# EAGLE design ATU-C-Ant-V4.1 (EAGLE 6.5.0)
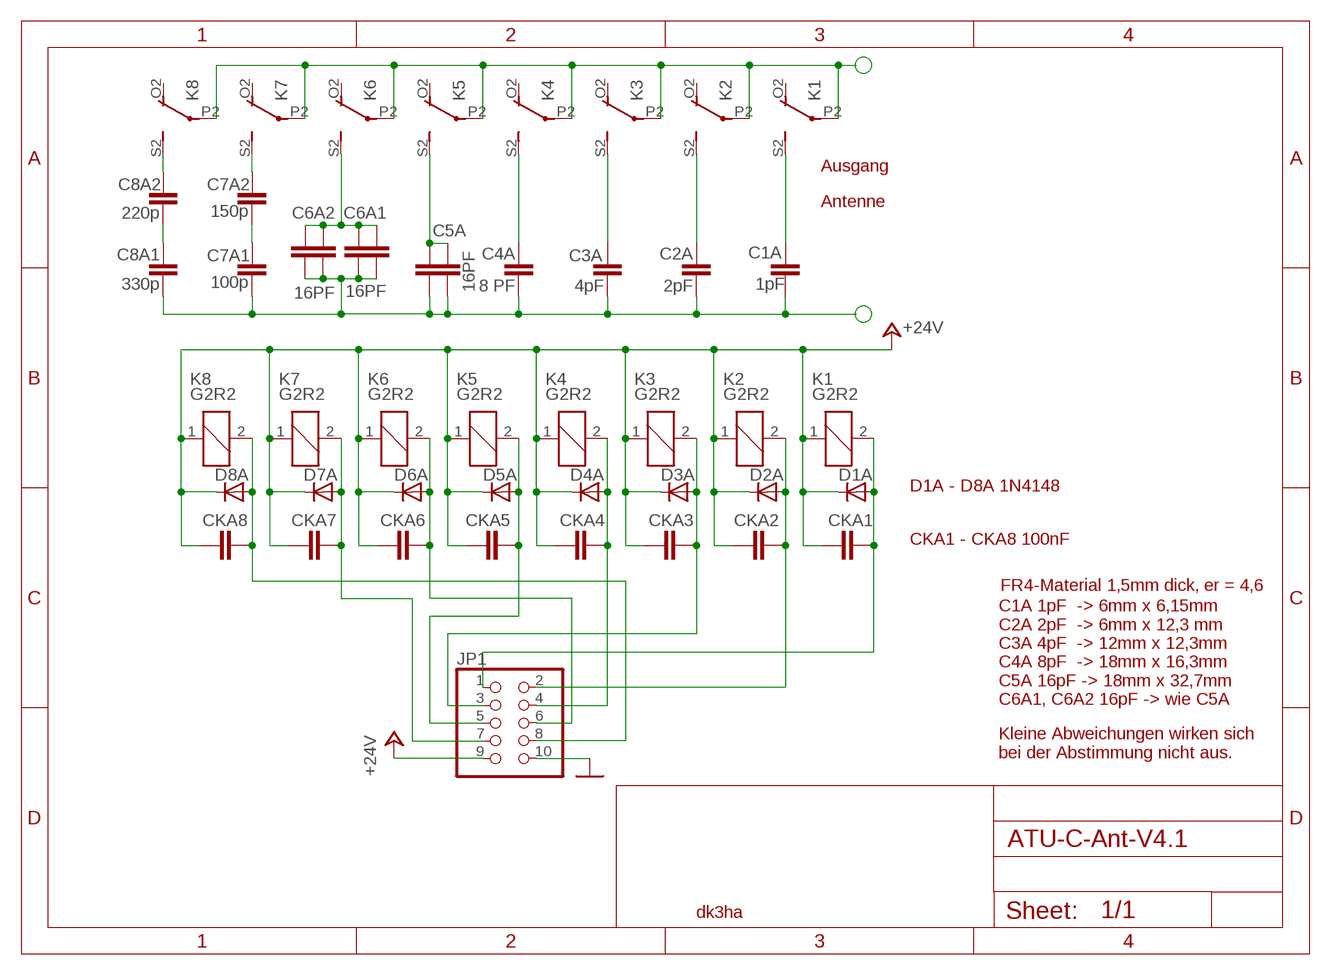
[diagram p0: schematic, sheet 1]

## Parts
C1A  1pF  1PF-CU-DS-ER4,6-D1,5  [1PF-ER4.6-DS-1,5]
C2A  2pF  2PF-CU-DS-ER4,6-D1,5  [2PF-ER4.6-DS-1,5]
C3A  4pF  4PF-CU-DS-ER4,6-D1,5  [4PF-ER4.6-DS-1,5]
C4A  8 PF  8PF-CU-DS-ER4,6-D1,5  [8PF-ER4.6-DS-1,5]
C5A  16PF  16PF-CU-DS-ER4,6-D1,5  [16PF-ER4.6-DS-1,5]
C6A1  16PF  16PF-CU-DS-ER4,6-D1,5  [16PF-ER4.6-DS-1,5]
C6A2  16PF  16PF-CU-DS-ER4,6-D1,5  [16PF-ER4.6-DS-1,5]
C7A1  100p  C15/5  [C15B5]
C7A2  150p  C15/5  [C15B5]
C8A1  330p  C15/5  [C15B5]
C8A2  220p  C15/5  [C15B5]
CKA1  C-EUC1206  [C1206]
CKA2  C-EUC1206  [C1206]
CKA3  C-EUC1206  [C1206]
CKA4  C-EUC1206  [C1206]
CKA5  C-EUC1206  [C1206]
CKA6  C-EUC1206  [C1206]
CKA7  C-EUC1206  [C1206]
CKA8  C-EUC1206  [C1206]
D1A  DIODE-MINIMELF  [MINIMELF]
D2A  DIODE-MINIMELF  [MINIMELF]
D3A  DIODE-MINIMELF  [MINIMELF]
D4A  DIODE-MINIMELF  [MINIMELF]
D5A  DIODE-MINIMELF  [MINIMELF]
D6A  DIODE-MINIMELF  [MINIMELF]
D7A  DIODE-MINIMELF  [MINIMELF]
D8A  DIODE-MINIMELF  [MINIMELF]
JP1  PINHD-2X5  [2X05]
K1  G2R2  [G2R2]
K2  G2R2  [G2R2]
K3  G2R2  [G2R2]
K4  G2R2  [G2R2]
K5  G2R2  [G2R2]
K6  G2R2  [G2R2]
K7  G2R2  [G2R2]
K8  G2R2  [G2R2]

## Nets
+24V: CKA1.1 CKA2.1 CKA3.1 CKA4.1 CKA5.1 CKA6.1 CKA7.1 CKA8.1 D1A.C D2A.C D3A.C D4A.C D5A.C D6A.C D7A.C D8A.C JP1.9 K1.1 K2.1 K3.1 K4.1 K5.1 K6.1 K7.1 K8.1
GND: JP1.10
LSP2: C1A.P$1 C2A.P$1 C3A.P$1 C4A.P$1 C5A.P$2 C5A.P$4 C6A1.P$2 C6A1.P$4 C6A2.P$2 C6A2.P$4 C7A1.2 C8A1.2
N$1: C6A1.P$1 C6A1.P$3 C6A2.P$1 C6A2.P$3 K6.S2(3:S)
N$3: C7A1.1 C7A2.1
N$4: C8A2.1 K8.S2(3:S)
N$5: C8A1.1 C8A2.2
N$6: C7A2.2 K7.S2(3:S)
N$7: C4A.P$2 K4.S2(3:S)
N$8: CKA1.2 D1A.A JP1.1 K1.2
N$9: K1.P2(3:P) K2.P2(3:P) K3.P2(3:P) K4.P2(3:P) K5.P2(3:P) K6.P2(3:P) K7.P2(3:P) K8.P2(3:P)
N$10: C3A.P$2 K3.S2(3:S)
N$11: CKA2.2 D2A.A JP1.2 K2.2
N$12: C2A.P$2 K2.S2(3:S)
N$13: CKA3.2 D3A.A JP1.3 K3.2
N$14: C1A.P$2 K1.S2(3:S)
N$15: CKA4.2 D4A.A JP1.4 K4.2
N$20: CKA6.2 D6A.A JP1.6 K6.2
N$22: C5A.P$1 C5A.P$3 K5.S2(3:S)
N$26: CKA7.2 D7A.A JP1.7 K7.2
N$28: CKA8.2 D8A.A JP1.8 K8.2
N$A5: CKA5.2 D5A.A JP1.5 K5.2
Unconnected: K1.O1(2:O) K1.O2(3:O) K1.P1(2:P) K1.S1(2:S) K2.O1(2:O) K2.O2(3:O) K2.P1(2:P) K2.S1(2:S) K3.O1(2:O) K3.O2(3:O) K3.P1(2:P) K3.S1(2:S) K4.O1(2:O) K4.O2(3:O) K4.P1(2:P) K4.S1(2:S) K5.O1(2:O) K5.O2(3:O) K5.P1(2:P) K5.S1(2:S) K6.O1(2:O) K6.O2(3:O) K6.P1(2:P) K6.S1(2:S) K7.O1(2:O) K7.O2(3:O) K7.P1(2:P) K7.S1(2:S) K8.O1(2:O) K8.O2(3:O) K8.P1(2:P) K8.S1(2:S)

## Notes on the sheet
- Ausgang
- Antenne
- D1A - D8A 1N4148
- CKA1 - CKA8 100nF
- FR4-Material 1,5mm dick, er = 4,6
- C1A 1pF  -> 6mm x 6,15mm
  C2A 2pF  -> 6mm x 12,3 mm
  C3A 4pF  -> 12mm x 12,3mm
  C4A 8pF  -> 18mm x 16,3mm
  C5A 16pF -> 18mm x 32,7mm
  C6A1, C6A2 16pF -> wie C5A
- Kleine Abweichungen wirken sich
  bei der Abstimmung nicht aus.
- dk3ha

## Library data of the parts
C1A = dk3ha-2020:1PF-CU-DS-ER4,6-D1,5: C doppelseitig Cu, d=1,5mm, Epoxy er=4,6 (Bungard), 1 pF, Maße 6,2mm x 6mm
C2A = dk3ha-2020:2PF-CU-DS-ER4,6-D1,5: C doppelseitig Cu, d=1,5mm, Epoxy er=4,6 (Bungard), 2 pF, Maße 12,3mm x 6mm
C3A = dk3ha-2020:4PF-CU-DS-ER4,6-D1,5: C doppelseitig Cu, d=1,5mm, Epoxy er=4,6 (Bungard), 4 pF, Maße 12,3mm x 12mm
C4A = dk3ha-2020:8PF-CU-DS-ER4,6-D1,5: C doppelseitig Cu, d=1,5mm, Epoxy er=4,6 (Bungard), 8 pF, Maße 16,4mm x 18mm
C5A C6A1 C6A2 = dk3ha-2020:16PF-CU-DS-ER4,6-D1,5: C doppelseitig Cu, d=1,5mm, Epoxy er=4,6 (Bungard), 16 pF, Maße 32,8mm x 18mm
C7A1 C7A2 C8A1 C8A2 = capacitor-wima:C: CAPACITOR
CKA1-CKA8 = rcl:C-EU: CAPACITOR, European symbol
D1A D2A D3A D4A D5A D6A D7A D8A = diode:DIODE-: DIODE
JP1 = pinhead+:PINHD-2X5: PIN HEADER
K1-K8 = relay:G2R2: RELAY 2 x switch, Omron; MF: OMRON COMPONENTS USA; MPN: G2R-2-DC6; OC_FARNELL: unknown; OC_NEWARK: 89C5317

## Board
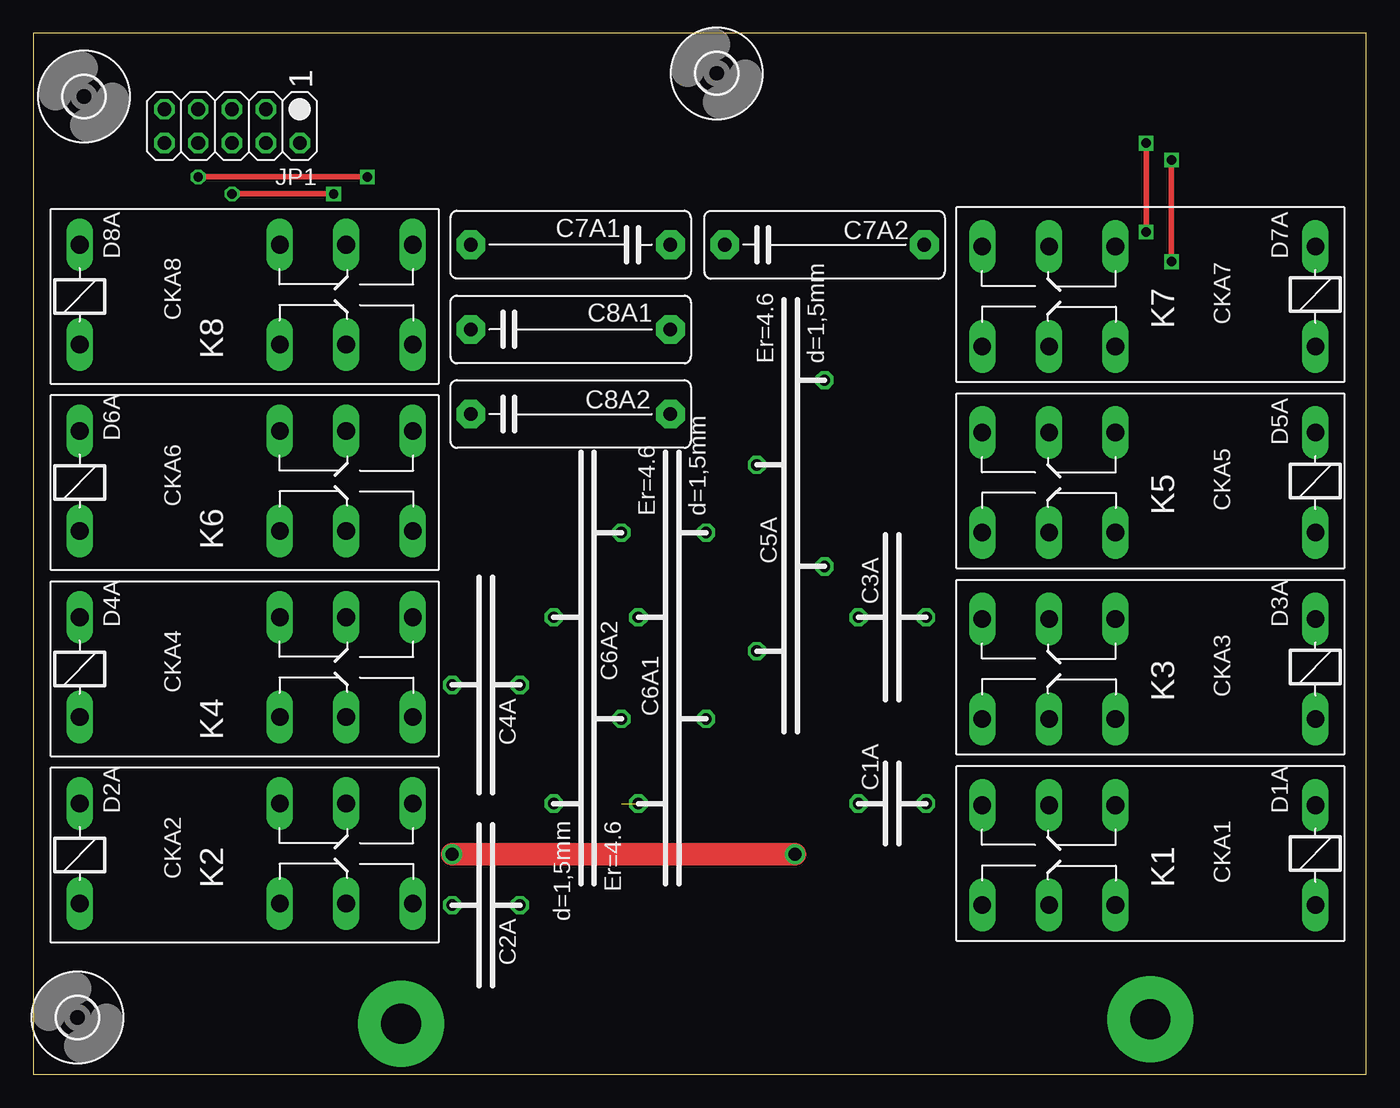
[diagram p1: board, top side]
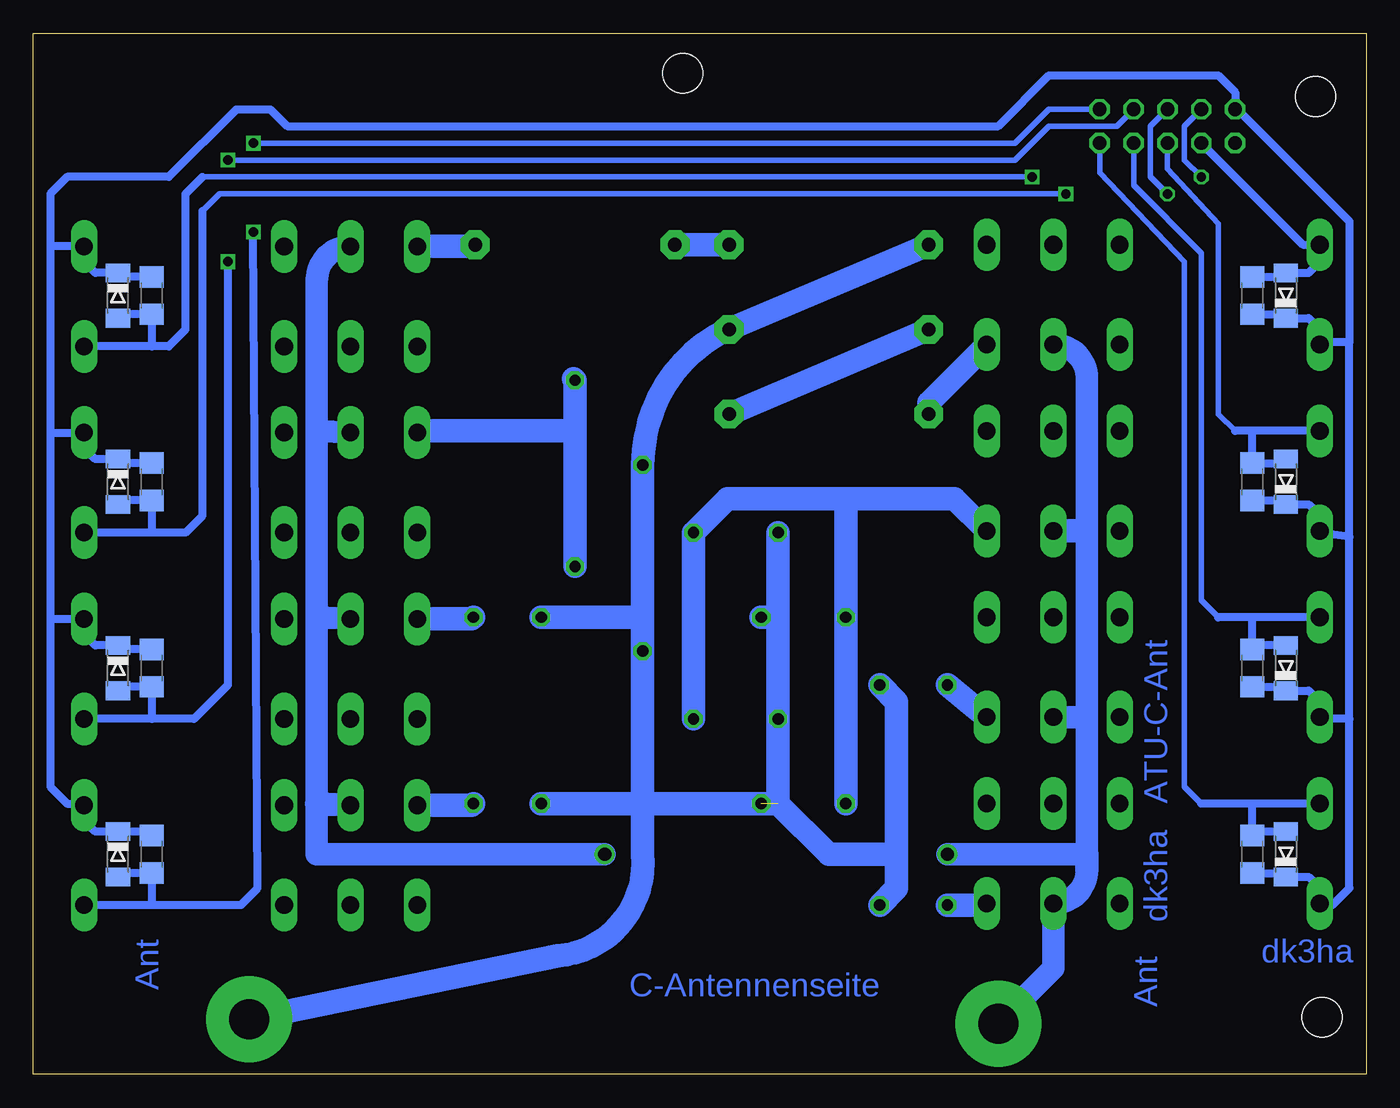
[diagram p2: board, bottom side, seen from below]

Size 100 x 78.08 mm. Coordinates in mm from the lower left corner, seen from the top.
Outline: 100,0 100,78.08 0,78.08 0,0 100,0
Copper layers (1*16): Top 0.035mm / dielectric 1.5mm / Bottom 0.035mm
Design rules "default": minimum track width 10mil, minimum drill 24mil, track to track 8mil, track to pad 8mil, pad to pad 8mil, via to via 8mil, smd to smd 8mil, copper to edge 40mil, drill to drill 8mil, minimum pad ring 10mil, minimum via ring 8mil, stop-mask expansion 4mil, vias tented up to drill 0mil, thermal gap 10mil

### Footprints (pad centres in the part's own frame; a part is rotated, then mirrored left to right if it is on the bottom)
1PF-ER4.6-DS-1,5 = drill 0.85 octagon: P$1 -2.54,0; P$2 2.54,0
2PF-ER4.6-DS-1,5 = drill 0.85 octagon: P$1 -2.54,0; P$2 2.54,0
4PF-ER4.6-DS-1,5 = drill 0.85 octagon: P$1 -2.54,0; P$2 2.54,0
8PF-ER4.6-DS-1,5 = drill 0.85 octagon: P$1 -2.54,0; P$2 2.54,0
16PF-ER4.6-DS-1,5 = drill 0.85 octagon: P$1 2.54,10.16; P$2 -2.54,3.81; P$3 2.54,-3.81; P$4 -2.54,-10.16
C15B5 = drill 1.016 pad 2.159 octagon: 1 -7.493,0; 2 7.493,0
C1206 = smd 1.6 x 1.8: 1 -1.4,0; 2 1.4,0
MINIMELF = smd 1.4 x 1.8: A 1.7,0; C -1.7,0
2X05 = drill 1.016 octagon: 1 -5.08,-1.27; 2 -5.08,1.27; 3 -2.54,-1.27; 4 -2.54,1.27; 5 0,-1.27; 6 0,1.27; 7 2.54,-1.27; 8 2.54,1.27; 9 5.08,-1.27; 10 5.08,1.27
G2R2 = drill 1.321 long: 1 -2.54,-3.683; 2 -2.54,3.81; O1 12.471,3.81; O2 12.471,-3.683; P1 17.45,3.81; P2 17.45,-3.683; S1 22.454,3.81; S2 22.454,-3.683
3,0 = hole 3: 0,0

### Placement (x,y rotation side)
C1A  64.44,20.32 0 top
C2A  33.96,12.7 180 top
C3A  64.44,34.29 0 top
C4A  33.96,29.21 180 top
C5A  56.82,41.91 0 top
C6A1  47.93,30.48 0 top
C6A2  41.58,30.48 180 top
C7A1  40.31,62.23 180 top
C7A2  59.36,62.23 0 top
C8A1  40.31,55.88 0 top
C8A2  40.31,49.53 0 top
CKA1  91.11,16.51 270 bottom
CKA2  8.56,16.51 90 bottom
CKA3  91.11,30.48 270 bottom
CKA4  8.56,30.48 90 bottom
CKA5  91.11,44.45 270 bottom
CKA6  8.56,44.45 90 bottom
CKA7  91.11,58.42 270 bottom
CKA8  8.56,58.42 90 bottom
D1A  93.65,16.51 270 bottom
D2A  6.02,16.51 90 bottom
D3A  93.65,30.48 270 bottom
D4A  6.02,30.48 90 bottom
D5A  93.65,44.45 270 bottom
D6A  6.02,44.45 90 bottom
D7A  93.65,58.42 270 bottom
D8A  6.02,58.42 90 bottom
JP1  14.91,71.12 180 top
K1  93.65,16.51 180 top
K2  6.02,16.51 0 top
K3  93.65,30.48 180 top
K4  6.02,30.48 0 top
K5  93.65,44.45 180 top
K6  6.02,44.45 0 top
K7  93.65,58.42 180 top
K8  6.02,58.42 0 top
U$1  [3,0]  3.8,73.34 90 top
U$2  [3,0]  3.32,4.29 90 top
U$3  [3,0]  51.26,75.09 90 top

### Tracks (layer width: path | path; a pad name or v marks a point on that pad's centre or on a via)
+24V
  Bottom 0.61: 98.73,34.16 K3.1 96.19,33.02 95.35,32.18 D3A.C 93.35,31.88 CKA3.1 | 98.73,48.13 K5.1 96.19,46.99 95.35,46.15 D5A.C 93.35,45.85 CKA5.1 | K2.1 3.48,12.7 | K4.1 3.48,26.67 | K6.1 3.48,40.64 | K8.1 3.48,54.61 | 1.26,26.67 1.26,13.97 2.53,12.7 3.61,12.7 K2.1 | 1.26,26.67 1.26,40.32 | 1.26,40.32 1.26,54.93 | 1.26,54.93 1.26,63.82 1.26,63.98 9.67,72.39 JP1.9 9.83,73.66 11.1,74.93 23.8,74.93 27.61,71.12 80.95,71.12 82.22,72.39 84.76,72.39 89.84,67.31 97.46,67.31 98.73,66.04 98.73,62.23 | 98.73,62.23 98.73,48.13 | 98.73,48.13 98.73,34.16 | 98.73,34.16 98.73,21.59 97.46,20.32 96.32,20.32 K1.1 96.19,19.05 95.35,18.21 D1A.C 91.11,18.21 CKA1.1 | 98.73,62.23 98.6,62.1 K7.1 96.19,60.96 95.35,60.12 D7A.C 93.35,59.82 CKA7.1 | 1.26,26.67 3.61,26.67 K4.1 | 1.26,40.32 3.61,40.64 K6.1 | 1.26,54.93 3.67,54.93 K8.1 | CKA2.1 6.32,15.11 D2A.C 4.32,14.81 3.48,13.97 K2.1 | CKA4.1 6.32,29.08 D4A.C 4.32,28.78 3.48,27.94 K4.1 | CKA6.1 6.32,43.05 D6A.C 4.32,42.75 3.48,41.91 K6.1 | CKA8.1 6.32,57.02 D8A.C 4.32,56.72 3.48,55.88 K8.1
LSP2  (via drill 3 pad 6.45)  (1 unrouted)
  Bottom 1.778: C1A.P$1 54.28,20.32 | C7A1.2 C8A1.2 47.93,55.88 arc-64 C5A.P$2 54.28,34.29 | 54.28,34.29 C5A.P$4 54.28,20.32 | C3A.P$1 54.28,34.29 | C4A.P$1 35.23,27.94 35.23,16.51 | 35.23,16.51 35.23,13.97 C2A.P$1 | C6A2.P$4 44.12,34.29 | 44.12,34.29 C6A2.P$2 44.12,20.32 | 44.12,20.32 40.31,16.51 35.23,16.51 | C6A1.P$2 44.12,34.29 | 54.28,20.32 44.12,20.32 | 54.28,20.32 54.28,16.51 arc90 60.63,8.89 v83.81,4.13
N$1
  Bottom 1.778: C6A1.P$3 C6A1.P$1 47.93,43.18 39.04,43.18 | 39.04,43.18 30.89,43.18 K6.S2 | 39.04,43.18 C6A2.P$3 C6A2.P$1
N$3
  Bottom 1.778: C7A1.1 C7A2.1
N$4
  Bottom 1.778: C8A2.1 32.82,50.39 K8.S2
N$5
  Bottom 1.778: C8A2.2 C8A1.1
N$6
  Bottom 1.778: K7.S2 67.11,62.1 66.98,62.23 C7A2.2
N$7
  Bottom 1.778: C4A.P$2 29.87,27.94 K4.S2
N$8  (via drill 0.7)
  Top 0.406: v83.49,63.18 v83.49,69.85
  Bottom 0.406: v83.49,69.85 26.34,69.85 23.8,72.39 JP1.1
  Bottom 0.61: v83.49,63.18 83.17,13.97 84.44,12.7 91.11,12.7 | 91.11,12.7 K1.2 | 91.11,12.7 CKA1.2 93.35,15.11 D1A.A
N$9  (via drill 1 pad 1.27, 3 pad 6.45)
  Top 1.676: v57.14,16.51 v31.42,16.51
  Bottom 1.524: 21.07,26.8 20.94,26.67 | 21.07,40.77 20.94,40.64 | K2.P2 23.67,12.83
  Bottom 1.676: K4.P2 21.07,26.8 | 78.73,48.26 78.73,59.58 arc90 K7.P2 | 78.73,48.26 78.73,34.29 | 78.73,34.29 78.73,20.32 78.73,16.51 v57.14,16.51 60.63,16.51 | v31.42,16.51 20.94,16.51 20.94,26.67 20.94,40.64 20.94,52.21 arc-90 K8.P2 | K3.P2 78.73,34.29 | K5.P2 78.73,48.26 | 20.94,15.35 arc90 K2.P2 23.47,7.95 v27.61,3.81
  Bottom 1.778: 20.94,16.51 20.94,15.35 | K6.P2 21.07,40.77 | K1.P2 78.73,20.32
N$10
  Bottom 1.778: K3.S2 67.11,34.16 C3A.P$2
N$11
  Bottom 0.406: JP1.2 19.99,67.63 13.64,60.96 13.64,21.59 12.37,20.32
  Bottom 0.61: K2.2 8.56,20.32 | 8.56,20.32 12.37,20.32 | 8.56,20.32 CKA2.2 8.26,18.21 D2A.A
N$12
  Bottom 1.778: C2A.P$2 28.6,12.7 K2.S2
N$13  (via drill 0.7)
  Top 0.406: v85.39,60.96 v85.39,68.58
  Bottom 0.406: v85.39,68.58 26.34,68.58 23.8,71.12 18.72,71.12 JP1.3
  Bottom 0.61: v85.39,60.96 85.39,29.21 87.94,26.67 91.11,26.67 | 91.11,26.67 K3.2 | 91.11,26.67 CKA3.2 93.35,29.08 D3A.A
N$14
  Bottom 1.778: K1.S2 67.11,20.19 C1A.P$2
N$15
  Bottom 0.406: 11.1,34.29 12.37,35.56 12.37,61.59 17.45,66.67 JP1.4
  Bottom 0.61: K4.2 8.56,34.29 | 8.56,34.29 11.1,34.29 | 8.56,34.29 CKA4.2 8.26,32.18 D4A.A
N$20
  Bottom 0.406: JP1.6 14.91,67.94 11.1,63.82 11.1,49.53 9.83,48.26
  Bottom 0.61: K6.2 8.56,48.26 | 8.56,48.26 9.83,48.26 | 8.56,48.26 CKA6.2 6.32,45.85 D6A.A
N$22
  Bottom 1.778: 59.49,52.2 C5A.P$1 59.36,48.26 | C5A.P$3 59.36,48.26 | K5.S2 71.2,48.26 59.36,48.26
N$26  (via drill 0.7)
  Top 0.406: v12.37,67.31 v25.07,67.31
  Bottom 0.406: JP1.7 13.64,71.12 13.64,68.58 v12.37,67.31 | v25.07,67.31 87.3,67.31
  Bottom 0.61: 87.3,67.31 88.57,66.04 88.57,55.88 89.84,54.61 91.11,54.61 | 91.11,54.61 K7.2 | 91.11,54.61 CKA7.2 93.35,57.02 D7A.A
N$28
  Bottom 0.61: JP1.8 4.75,62.23 K8.2 3.48,60.96 4.32,60.12 D8A.A 6.32,59.82 CKA8.2
N$A5  (via drill 0.7)
  Top 0.406: v22.53,66.04 v14.91,66.04
  Bottom 0.406: 87.3,64.77 86.03,66.04 v22.53,66.04 | v14.91,66.04 16.18,67.31 16.18,71.12 JP1.5
  Bottom 0.61: 87.3,64.77 87.3,41.91 88.57,40.64 91.11,40.64 | 91.11,40.64 K5.2 | 91.11,40.64 CKA5.2 93.35,43.05 D5A.A

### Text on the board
Bottom: ATU-C-Ant | dk3ha | dk3ha | Ant | Ant | C-Antennenseite
tPlace: 1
